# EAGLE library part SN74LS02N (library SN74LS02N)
QUADRUPLE 2-INPUT POSITIVE-NOR GATES Source: Datasheet
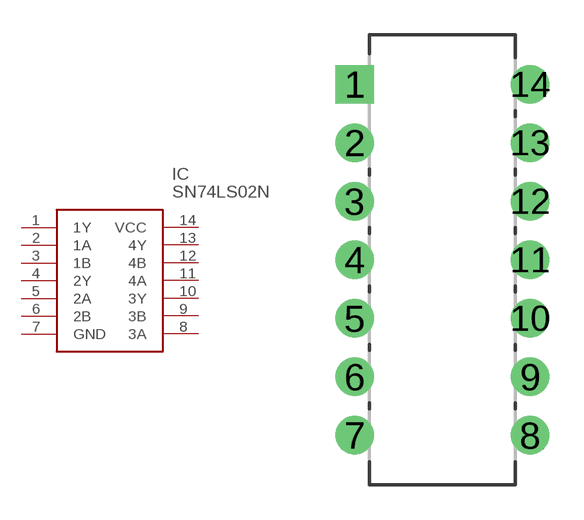
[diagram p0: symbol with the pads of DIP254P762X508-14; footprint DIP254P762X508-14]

Designator prefix IC

## SN74LS02N (Description: QUADRUPLE 2-INPUT POSITIVE-NOR GATES; Height: mm; Manufacturer_Name: Texas Instruments; Manufacturer_Part_Number: SN74LS02N; Mouser_Part_Number: 595-SN74LS02N; Mouser_Price-Stock: https://www.mouser.com/Search/Refine.aspx?Keyword=595-SN74LS02N; RS_Part_Number: 3685907; RS_Price-Stock: http://uk.rs-online.com/web/p/products/3685907)  [DIP254P762X508-14]
1  1Y
2  1A
3  1B
4  2Y
5  2A
6  2B
7  GND
8  3A
9  3B
10  3Y
11  4A
12  4B
13  4Y
14  VCC

## Footprint DIP254P762X508-14 (pad centres in mm)
DIP254P762X508-14
drill 1.118 pad 1.676 square: 1 -7.62,15.24
drill 1.118 pad 1.676: 2 -7.62,12.7; 3 -7.62,10.16; 4 -7.62,7.62; 5 -7.62,5.08; 6 -7.62,2.54; 7 -7.62,0; 8 0,0; 9 0,2.54; 10 0,5.08; 11 0,7.62; 12 0,10.16; 13 0,12.7; 14 0,15.24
